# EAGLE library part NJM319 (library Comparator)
NJM319 高速コンパレータ datasheet
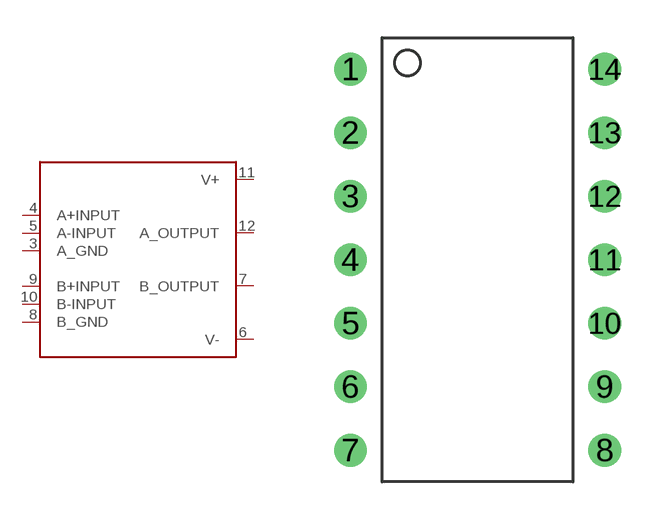
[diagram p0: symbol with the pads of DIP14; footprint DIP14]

Designator prefix -

## NJM319U  [DIP14]
3  A_GND
4  A+INPUT
5  A-INPUT
6  V-
7  B_OUTPUT
8  B_GND
9  B+INPUT
10  B-INPUT
11  V+
12  A_OUTPUT

## Footprint DIP14 (pad centres in mm)
DIPパッケージ 14ピン
drill 0.8: 1 -5.08,7.62; 2 -5.08,5.08; 3 -5.08,2.54; 4 -5.08,0; 5 -5.08,-2.54; 6 -5.08,-5.08; 7 -5.08,-7.62; 8 5.08,-7.62; 9 5.08,-5.08; 10 5.08,-2.54; 11 5.08,0; 12 5.08,2.54; 13 5.08,5.08; 14 5.08,7.62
